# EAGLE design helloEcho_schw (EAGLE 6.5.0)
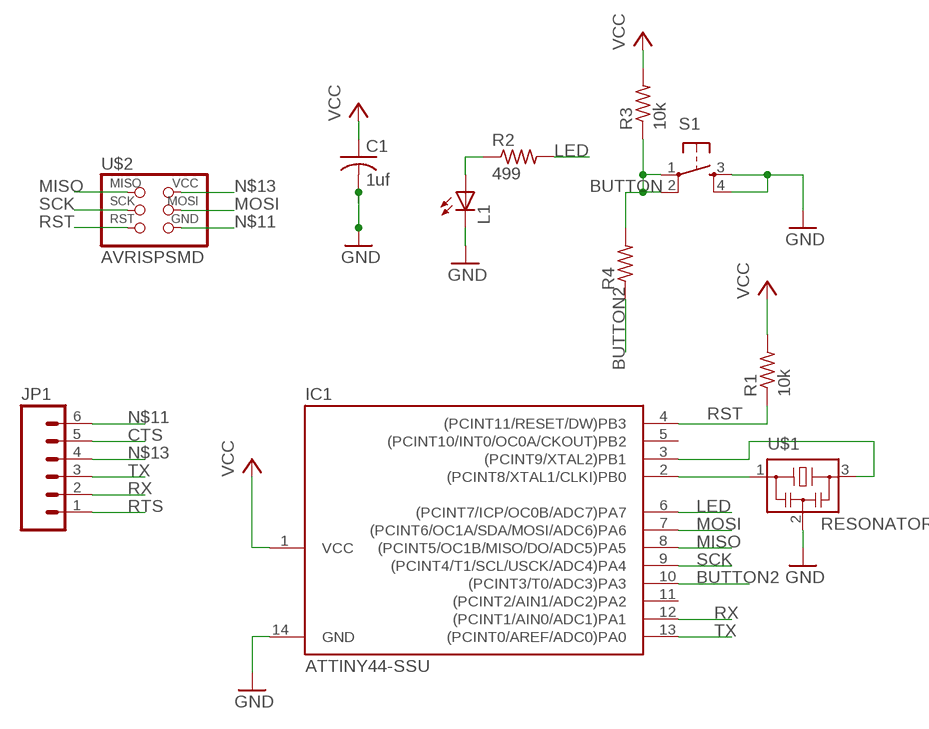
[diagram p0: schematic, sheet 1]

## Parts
C1  1uf  C-USC1206  [C1206]
IC1  ATTINY44-SSU  [SOIC14]
JP1  M06SMD  [1X06-SMD]
L1  LED1206  [1206]
R1  10k  R-US_R1206  [R1206]
R2  499  RESISTOR1206  [1206]
R3  10k  RESISTOR1206  [1206]
R4  RESISTOR1206  [1206]
S1  6MM_SWITCH6MM_SWITCH  [6MM_SWITCH]
U$1  RESONATOR  [EFOBM]
U$2  AVRISPSMD  [2X03SMD]

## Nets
BUTTON: R3.1 R4.2 S1.1(P) S1.2(P1)
BUTTON2: IC1.10((PCINT3/T0/ADC3)PA3) R4.1
CTS: JP1.5
LED: IC1.6((PCINT7/ICP/OC0B/ADC7)PA7) R2.2
MISO: IC1.8((PCINT5/OC1B/MISO/DO/ADC5)PA5) U$2.1(MISO)
MOSI: IC1.7((PCINT6/OC1A/SDA/MOSI/ADC6)PA6) U$2.4(MOSI)
N$1: IC1.2((PCINT8/XTAL1/CLKI)PB0) U$1.1
N$2: IC1.3((PCINT9/XTAL2)PB1) U$1.3
N$3: L1.1(A) R2.1
N$11: C1.2 IC1.14(GND) JP1.6 L1.2(C) S1.3(S) S1.4(S1) U$1.2 U$2.6(GND) ; supply symbol labelled GND
N$13: C1.1 IC1.1(VCC) JP1.4 R1.2 R3.2 U$2.2(VCC) ; supply symbol labelled VCC
RST: IC1.4((PCINT11/RESET/DW)PB3) R1.1 U$2.5(RST)
RTS: JP1.1
RX: IC1.12((PCINT1/AIN0/ADC1)PA1) JP1.2
SCK: IC1.9((PCINT4/T1/SCL/USCK/ADC4)PA4) U$2.3(SCK)
TX: IC1.13((PCINT0/AREF/ADC0)PA0) JP1.3
Unconnected: IC1.5((PCINT10/INT0/OC0A/CKOUT)PB2) IC1.11((PCINT2/AIN1/ADC2)PA2)

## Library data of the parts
C1 = rcl:C-US: CAPACITOR, American symbol
IC1 = fab:ATTINY44
JP1 = SparkFun:M06: Header 6 Standard 6-pin 0.1" header. Use with straight break away headers (SKU : PRT-00116), right angle break away headers (PRT-00553), swiss pins (PRT-00743), machine pins (PRT-00117), and female headers (PRT-00115). Molex polarized connector foot print use with SKU : PRT-08094 with associated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
L1 = 01_FAB_Hello:LED
R1 = resistor:R-US_: RESISTOR, American symbol
R2 R3 = 01_ng:RESISTOR
R4 = 01_FAB_Hello:RESISTOR
S1 = 01_fab:6MM_SWITCH: OMRON SWITCH
U$1 = fab:RESONATOR
U$2 = fab:AVRISP

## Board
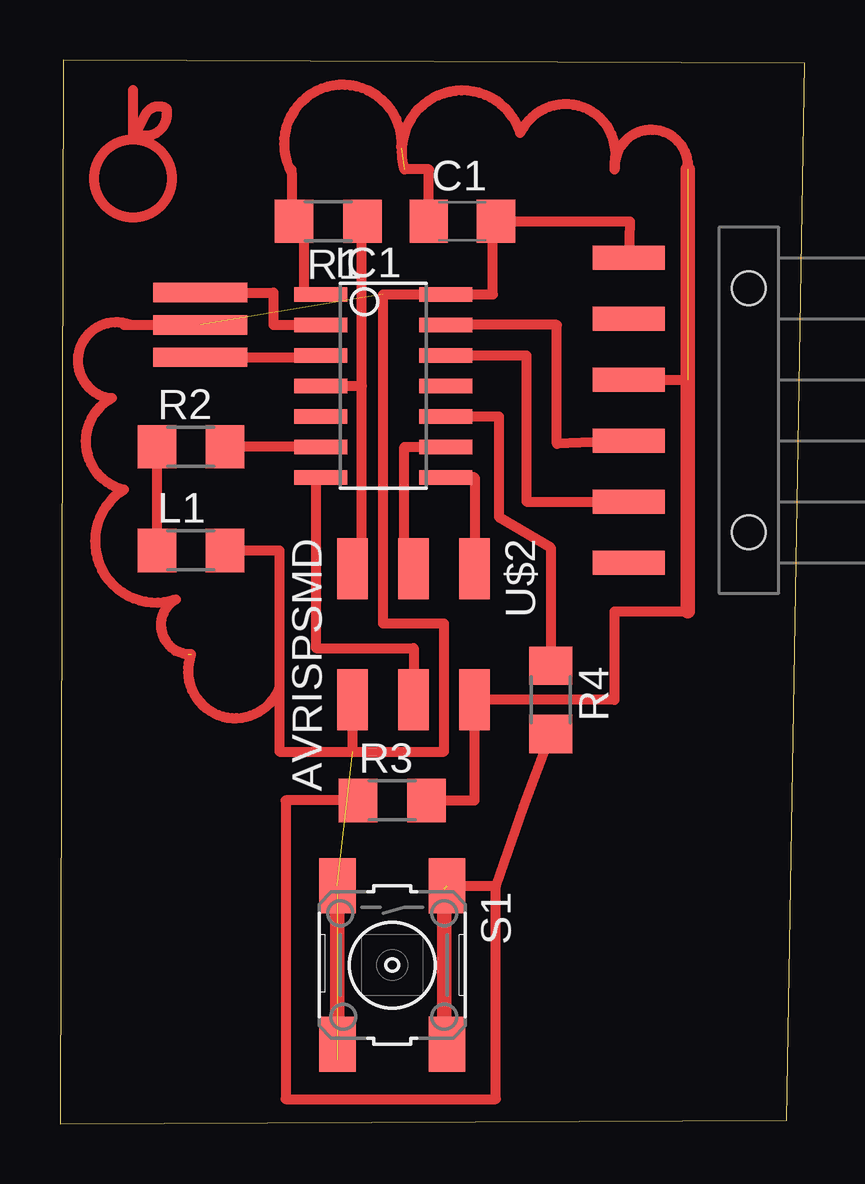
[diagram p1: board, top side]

Size 31.04 x 44.31 mm. Coordinates in mm from the lower left corner, seen from the top.
Outline: 0,0 30.28,0.13 31.04,44.19 0.13,44.31 0,0
Copper layers 1: Top 0.035mm
Design rules "ERP-1sided-10mil-16mill": minimum track width 10mil, minimum drill 24mil, track to track 16mil, track to pad 16mil, pad to pad 16mil, via to via 16mil, smd to smd 0mil, copper to edge 16mil, drill to drill 36mil, minimum pad ring 10mil, minimum via ring 8mil, stop-mask expansion 4mil, vias tented up to drill 0mil, thermal gap 10mil

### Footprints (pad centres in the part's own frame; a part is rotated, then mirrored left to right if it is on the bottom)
C1206 = smd 1.6 x 1.8: 1 -1.4,0; 2 1.4,0
SOIC14 = smd 0.61 x 2.21: 1 -3.81,-2.603; 2 -2.54,-2.603; 3 -1.27,-2.603; 4 0,-2.603; 5 1.27,-2.603; 6 2.54,-2.603; 7 3.81,-2.603; 8 3.81,2.603; 9 2.54,2.603; 10 1.27,2.603; 11 0,2.603; 12 -1.27,2.603; 13 -2.54,2.603; 14 -3.81,2.603
1X06-SMD = smd 1 x 3: 1 -6.35,5; 2 -3.81,5; 3 -1.27,5; 4 1.27,5; 5 3.81,5; 6 6.35,5 | hole 1.4: -5.08,0; 5.08,0
1206 = smd 1.6 x 1.803: 1 -1.422,0; 2 1.422,0
R1206 = smd 1.6 x 1.803: 1 -1.422,0; 2 1.422,0
6MM_SWITCH = smd 2.286 x 1.524: 1 -3.302,2.286; 2 3.302,2.286; 3 -3.302,-2.286; 4 3.302,-2.286
EFOBM = smd 0.8 x 3.9: 1 -1.35,0; 2 0,0; 3 1.35,0
2X03SMD = smd 2.54 x 1.27: 1 -2.54,2.54; 2 2.92,2.54; 3 -2.54,0; 4 2.92,0; 5 -2.54,-2.54; 6 2.92,-2.54

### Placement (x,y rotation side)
C1  16.76,37.59 0 top
IC1  13.46,30.73 270 top
JP1  28.7,29.72 90 top
L1  5.46,23.88 0 top
R1  11.18,37.59 180 top
R2  5.46,28.19 0 top
R3  13.84,13.46 0 top
R4  20.45,17.65 270 top
S1  13.84,6.6 270 top
U$1  5.84,33.27 270 top
U$2  14.73,20.57 270 top

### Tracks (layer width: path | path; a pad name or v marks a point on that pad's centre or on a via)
BUTTON  (1 unrouted)
  Top 0.406: R3.1 9.4,13.46 9.4,1.02 18.16,1.02 18.16,9.91 | S1.1 18.16,9.91 | R4.2 19.3,13.21 18.16,9.91
  Top 0.61: S1.2 16,3.3 16,9.78
BUTTON2
  Top 0.406: IC1.10 18.29,29.46 18.29,25.27 20.45,24 R4.1
LED
  Top 0.406: IC1.6 R2.2
MISO
  Top 0.406: IC1.8 17.27,26.92 U$2.1
MOSI
  Top 0.406: IC1.7 10.67,26.92 10.67,19.81 14.73,19.81 U$2.4
N$1
  Top 0.406: U$1.1 8.89,34.62 8.89,33.27 IC1.2
N$2
  Top 0.406: U$1.3 10.86,31.92 IC1.3
N$3
  Top 0.406: R2.1 L1.1
N$6
  Top 0.406: 2.92,33.27 arc190 2.03,30.23
N$10
  Top 0.406: 2.16,30.23 arc139 2.67,26.42 arc167 4.83,21.84
N$11  (3 unrouted)
  Top 0.406: 4.83,21.84 arc146 5.33,19.56 | 12.19,15.49 16,15.49 16,20.83 13.46,20.83 13.46,34.54 IC1.14 18.03,34.54 18.03,37.59 C1.2 23.75,37.59 JP1.6 | 2.67,33.27 U$1.2 | 12.19,15.49 U$2.6 | L1.2 9.14,23.88 9.14,18.16 | 9.14,18.16 9.14,15.49 12.19,15.49 | 5.46,19.56 arc180 9.14,18.16
  Top 0.61: S1.3 S1.4
N$13  (2 unrouted)
  Top 0.406: 23.11,40.01 arc165 19.18,41.28 arc180 14.35,39.75 15.37,39.75 C1.1 15.36,39.75 | 9.65,39.62 9.65,37.59 R1.2 10.16,37.59 10.16,34.54 IC1.1 | 9.65,39.62 9.65,39.75 | R3.2 17.27,13.46 U$2.2 23.11,17.65 23.11,21.34 26.16,21.34 | JP1.4 26.16,30.99 | 26.16,39.75 arc180 23.11,40.01 | 23.11,40.01 arc10 23.11,39.75 | 14.22,40.64 arc214 9.65,39.62
  Top 0.61: 26.16,39.75 26.16,21.34
N$16
  Top 0.406: 3.05,41.02 3.56,42.04 arc-95 4.45,42.29 4.45,42.04 arc-90 3.56,41.15 3.05,41.15 3.05,43.05
N$17  (1 unrouted)
RST
  Top 0.406: R1.1 12.57,37.59 12.57,30.73 | IC1.4 12.57,30.73 | U$2.5 12.57,23.11 12.57,30.73
RX
  Top 0.406: IC1.12 19.43,32 19.43,25.91 JP1.2
SCK
  Top 0.406: U$2.3 14.35,23.11 14.35,28.19 IC1.9
TX
  Top 0.406: JP1.3 20.7,28.32 20.7,33.27 IC1.13
(copper drawn outside any net)
  shapes: Top circle x1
